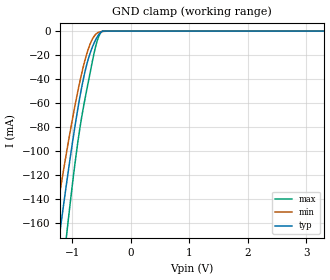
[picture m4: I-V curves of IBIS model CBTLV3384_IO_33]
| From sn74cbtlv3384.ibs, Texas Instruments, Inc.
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[Model]   CBTLV3384_IO_33
Model_type  Terminator
| variable   typ   min   max
C_comp   10pF   NA   NA
| C_tri-state   5.13pF   4.28pF   5.84pF
[Temperature Range]   40   100   -40
| Ambient temperature   25   85   -40
[Voltage range]   3.3   3   3.6
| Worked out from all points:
|   GND clamp passes 1 mA (typ) near -0.51 V on its own axis
[GND Clamp]
| CBTLV3384_IO_33
|   Voltage   I(typ)   I(min)   I(max)
-3.3V     -1.052A    -867.1mA   -1.329A
-1.31V    -205.6mA   -165.5mA   -269.7mA
-1.21V    -168.1mA   -134.7mA   -222.4mA
-1.095V   -126.8mA   -100.9mA   -170.2mA
-1.07V    -118.2mA   -93.87mA   -159.2mA
-915mV    -68.34mA   -53.08mA   -96.91mA
-800mV    -38.11mA   -27.84mA   -61.59mA
-675mV    -15.97mA   -8.815mA   -30.35mA
-605mV    -7.869mA   -3.113mA   -14.12mA
-555mV    -3.541mA   -1.115mA   -5.767mA
-475mV    -72.05uA   -328.9uA   -50.52uA
3.3V      1.318nA    61.76nA    17.29pA
